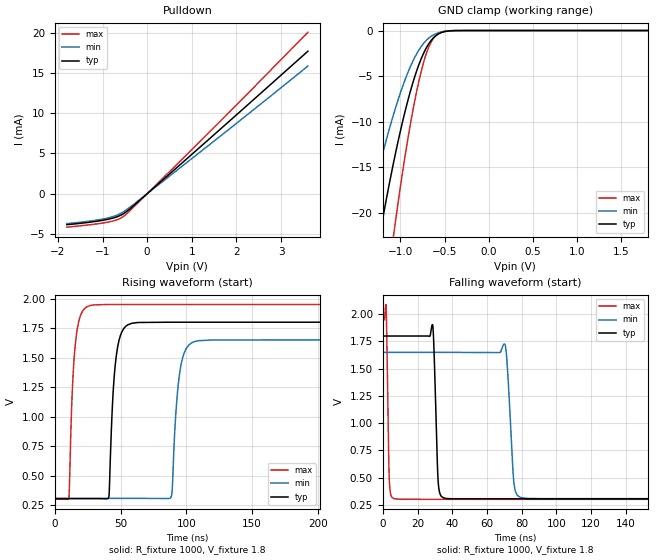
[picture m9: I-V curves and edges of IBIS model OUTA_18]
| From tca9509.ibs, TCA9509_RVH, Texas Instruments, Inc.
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[Model]   OUTA_18
Model_type  Open_drain
Enable   Active-High
Vref =   1.8
Rref =   1350
Cref =   50p
Vmeas =   0.9
| variable   typ   min   max
C_comp   2.28pF   1.60pF   2.61pF
| C_pulldown   1.51pF   1.09pF   1.75pF
| C_tri-state   2.28pF   1.60pF   2.61pF
[Temperature Range]   40   100   -40
| Ambient temperature   25   85   -40
[Voltage range]   1.8   1.65   1.95
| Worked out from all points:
|   slope of the pulldown table from 0 to 0.27 V, typ, clamps not added: 205 ohm
|   GND clamp passes 1 mA (typ) near -0.64 V on its own axis
|   rising waveform, R_fixture 1000, V_fixture 1.8: 20-80 % time 4.51ns typ, 5.09ns min, 4.03ns max; typ from 0.306 V to 1.8 V
|   falling waveform, R_fixture 1000, V_fixture 1.8: 20-80 % time 1.65ns typ, 2.67ns min, 1.01ns max; typ from 1.8 V to 0.306 V
[GND Clamp]
| OUTA_18
|   Voltage   I(typ)   I(min)   I(max)
-1.8V     -59.64mA   -41.37mA   -89.21mA
-1.415V   -33.14mA   -22.29mA   -50.68mA
-1.395V   -31.9mA    -21.4mA    -48.83mA
-1.23V    -22.27mA   -14.61mA   -34.37mA
-1.075V   -14.36mA   -9.116mA   -22.29mA
-950mV    -8.97mA    -5.465mA   -13.91mA
-830mV    -4.822mA   -2.801mA   -7.317mA
-730mV    -2.33mA    -1.324mA   -3.216mA
-645mV    -1.001mA   -587.8uA   -1.128mA
-555mV    -301.1uA   -202.9uA   -250.9uA
-430mV    -31.71uA   -30.66uA   -13.57uA
1.8V      507.9pA    2.612nA    99.77pA
[Pulldown]
| OUTA_18
|   Voltage   I(typ)   I(min)   I(max)
-1.8V     -3.852mA   -3.719mA   -4.16mA
-925mV    -3.233mA   -3.073mA   -3.582mA
-670mV    -2.859mA   -2.648mA   -3.228mA
-505mV    -2.396mA   -2.153mA   -2.713mA
1.48V     7.24mA     6.461mA    8.133mA
3.6V      17.7mA     15.87mA    20.05mA
[Ramp]
| OUTA_18
| variable   typ   min   max
dV/dt_r   0.90/4.49E-09   0.81/5.07E-09   0.99/4.03E-09
dV/dt_f   0.96/1.77E-09   0.85/2.84E-09   1.07/1.09E-09
R_load = 1000
[Rising Waveform]
| OUTA_18
R_fixture =   1000
C_fixture =   0
L_fixture =   0
V_fixture =   1.8
V_fixture_min = 1.65
V_fixture_max = 1.95
|   Time   V(typ)   V(min)   V(max)
0s        305.9mV    307.6mV    301.4mV
10.69ns   305.9mV    307.6mV    306.2mV
15.62ns   305.9mV    307.6mV    1.612V
25.03ns   305.9mV    307.6mV    1.934V
41.09ns   318.8mV    307.6mV    1.95V
46.22ns   1.463V     307.6mV    1.95V
55.55ns   1.778V     307.6mV    1.95V
88.51ns   1.8V       321.3mV    1.95V
104ns     1.8V       1.625V     1.95V
263.4ns   1.8V       1.65V      1.95V
[Falling Waveform]
| OUTA_18
R_fixture =   1000
C_fixture =   0
L_fixture =   0
V_fixture =   1.8
V_fixture_min = 1.65
V_fixture_max = 1.95
|   Time   V(typ)   V(min)   V(max)
0s        1.8V       1.65V      1.95V
1.861ns   1.8V       1.65V      2.074V
3.781ns   1.8V       1.65V      471.2mV
6.469ns   1.8V       1.65V      307.4mV
28.68ns   1.904V     1.65V      301.5mV
31.88ns   469.5mV    1.65V      301.5mV
35.08ns   314.3mV    1.65V      301.5mV
70.34ns   305.9mV    1.723V     301.5mV
79.23ns   305.9mV    319.3mV    301.5mV
263.4ns   305.9mV    307.6mV    301.4mV
